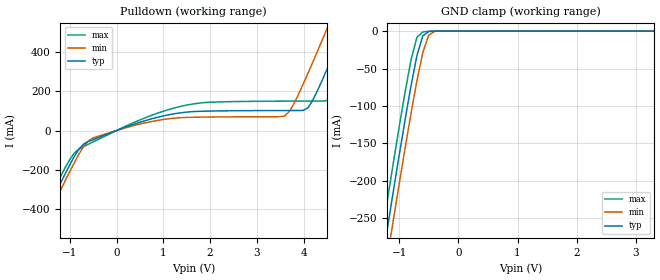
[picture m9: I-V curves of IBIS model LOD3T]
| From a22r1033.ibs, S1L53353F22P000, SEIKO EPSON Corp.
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[Model]   LOD3T
Model_type   Output
Polarity   Non-Inverting
|   typ   min   max
C_comp   5.0pF   4.0pF   6.0pF
|   typ   min   max
[Voltage range]   3.3   3.0   3.6
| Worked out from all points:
|   slope of the pulldown table from 0 to 0.495 V, typ, clamps not added: 11.9 ohm
|   GND clamp passes 1 mA (typ) near -0.51 V on its own axis
[Pulldown]
|   Voltage   I(typ)   I(min)   I(max)
-3.3V     -1.344A    -1.379A    -1.31A
-1.8V     -570.3mA   -607.2mA   -534.3mA
-1.7V     -519.4mA   -556.3mA   -483.4mA
-1V       -174.7mA   -209.1mA   -147.9mA
-500mV    -46.31mA   -38mA      -57.88mA
1.4V      91.11mA    65.79mA    124.5mA
3.6V      101.9mA    74.43mA    149.6mA
4.1V      117mA      294.2mA    149.9mA
4.5V      310.6mA    517.7mA    152.7mA
4.9V      535.5mA    746.5mA    330mA
5.3V      765.5mA    977.5mA    556mA
6.6V      1.523A     1.735A     1.313A
[GND_clamp]
|   Voltage   I(typ)   I(min)   I(max)
-3.3V     -1.343A    -1.379A    -1.309A
-1.3V     -314.1mA   -352.4mA   -276.2mA
-1.2V     -264.1mA   -302.5mA   -226.1mA
-1.1V     -214.6mA   -253.1mA   -176.6mA
-1V       -165.9mA   -204.2mA   -128.1mA
-900mV    -118.4mA   -156.3mA   -81.33mA
-800mV    -73.08mA   -109.9mA   -38.6mA
-700mV    -32.75mA   -66.18mA   -8.318mA
-600mV    -6.318mA   -28.41mA   -1.129mA
-500mV    -586.9uA   -5.399mA   -239.5uA
-400mV    -56.77uA   -404.4uA   -18.72uA
3.3V      7.178nA    15.7uA     6.022nA
[Ramp]
|   V_typ   V_min   V_max
dV/dt_r   1.98/0.84n   1.80/1.16n   2.16/0.61n
dV/dt_f   1.98/0.66n   1.80/0.91n   2.16/0.45n
R_load = 5000
